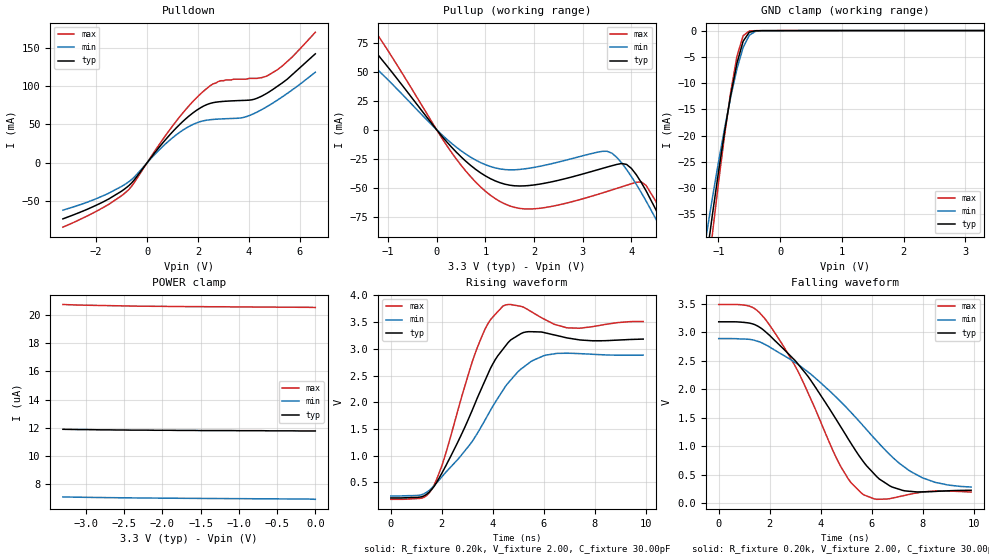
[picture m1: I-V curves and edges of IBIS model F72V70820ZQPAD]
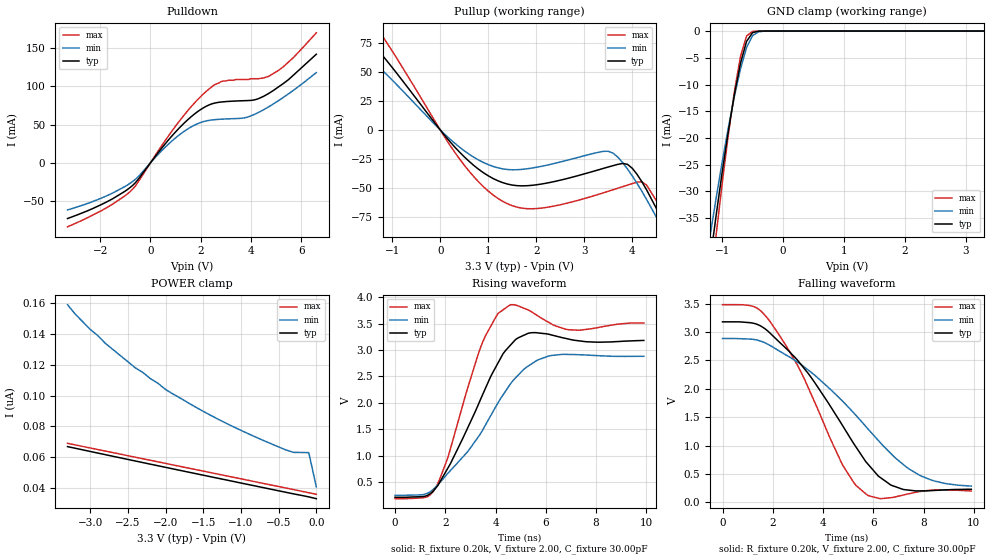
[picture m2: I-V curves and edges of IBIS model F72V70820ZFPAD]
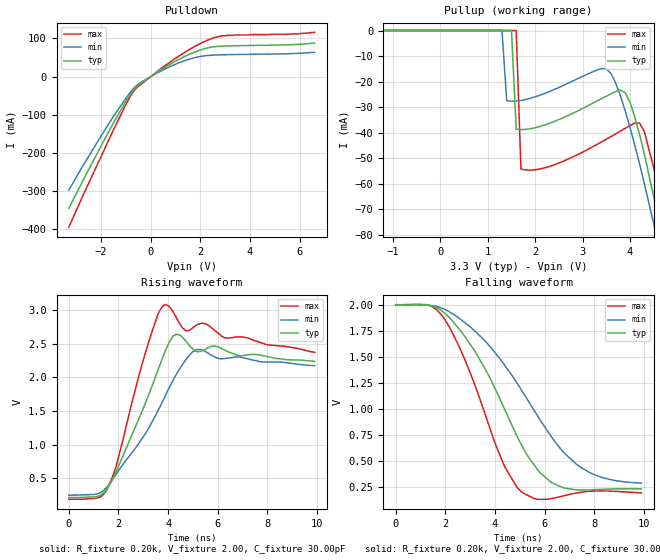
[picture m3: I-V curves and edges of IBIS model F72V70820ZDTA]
| IBIS file f72v7082.ibs created by s2ibis2 version 1.1
| North Carolina State University Electronics Research Laboratory  1995
[IBIS ver]   2.1
[File name]   f72v7082.ibs
[File Rev]   1.0
[Date]   02/03/2000
[Source]   Integrated Device Technology, Inc.
[Notes]   1. Temperatures: typ=25C, min=85C, max=-40C 2. Cemos9_3v
   process. 3. Ramp rates based on 50 ohm load.
[Copyright]   Copyright 1999, Integrated Device Technology, Inc.
|   Component idt72v70820z
[Component]   idt72v70820z
[Manufacturer]   Integrated Device Technology
[Package]
| variable   typ   min   max
R_pkg   0.75   0.60   0.90
L_pkg   8.10nH   8.30nH   9.90nH
C_pkg   0.53pF   0.46pF   0.60pF
[Pin]  signal_name   model_name   R_pin   L_pin   C_pin
1   GND   GND
2   VCC   POWER
3   TX8   F72V70820ZFPAD
4   TX9   F72V70820ZFPAD
5   TX10   F72V70820ZFPAD
6   TX11   F72V70820ZFPAD
7   TX12   F72V70820ZFPAD
8   TX13   F72V70820ZFPAD
9   TX14   F72V70820ZFPAD
10   TX15   F72V70820ZFPAD
11   GND   GND
12   RX0   F72V70820ZTTL2
13   RX1   F72V70820ZTTL2
14   RX2   F72V70820ZTTL2
15   RX3   F72V70820ZTTL2
16   RX4   F72V70820ZTTL2
17   RX5   F72V70820ZTTL2
18   RX6   F72V70820ZTTL2
19   RX7   F72V70820ZTTL2
20   RX8   F72V70820ZTTL2
21   RX9   F72V70820ZTTL2
22   RX10   F72V70820ZTTL2
23   RX11   F72V70820ZTTL2
24   RX12   F72V70820ZTTL2
25   RX13   F72V70820ZTTL2
26   RX14   F72V70820ZTTL2
27   RX15   F72V70820ZTTL2
28   F0I   F72V70820ZTTL
29   FE_HCLK   F72V70820ZTTL
30   GND   GND
31   CLK   F72V70820ZTTL
32   VCC   POWER
33   TMS   F72V70820ZTTLPU
34   TDI   F72V70820ZTTLPU
35   TDO   F72V70820ZFPAD
36   TCK   F72V70820ZTTL
37   TRST   F72V70820ZTTLU2
38   IC   F72V70820ZTTLPD
39   RESET   F72V70820ZTTL
40   WFPS   F72V70820ZTTL
41   A0   F72V70820ZTTL
42   A1   F72V70820ZTTL
43   A2   F72V70820ZTTL
44   A3   F72V70820ZTTL
45   A4   F72V70820ZTTL
46   A5   F72V70820ZTTL
47   A6   F72V70820ZTTL
48   A7   F72V70820ZTTL
49   DS_RD   F72V70820ZTTL
50   R_W_RW   F72V70820ZTTL
51   CS   F72V70820ZTTL
52   AS_ALE   F72V70820ZTTL
53   IM   F72V70820ZTTL
54   GND   GND
55   AD0   F72V70820ZQPAD
56   AD1   F72V70820ZQPAD
57   AD2   F72V70820ZQPAD
58   AD3   F72V70820ZQPAD
59   AD4   F72V70820ZQPAD
60   AD5   F72V70820ZQPAD
61   AD6   F72V70820ZQPAD
62   AD7   F72V70820ZQPAD
63   VCC   POWER
64   GND   GND
65   D8   F72V70820ZQPAD
66   D9   F72V70820ZQPAD
67   D10   F72V70820ZQPAD
68   D11   F72V70820ZQPAD
69   D12   F72V70820ZQPAD
70   D13   F72V70820ZQPAD
71   D14   F72V70820ZQPAD
72   D15   F72V70820ZQPAD
73   DTA   F72V70820ZDTA
74   CCO   F72V70820ZFPAD
75   GND   GND
76   ODE   F72V70820ZTTL
77   TX0   F72V70820ZFPAD
78   TX1   F72V70820ZFPAD
79   TX2   F72V70820ZFPAD
80   TX3   F72V70820ZFPAD
81   TX4   F72V70820ZFPAD
82   TX5   F72V70820ZFPAD
83   TX6   F72V70820ZFPAD
84   TX7   F72V70820ZFPAD
| Models and submodels in the file (8): F72V70820ZQPAD (I/O), F72V70820ZFPAD (3-state), F72V70820ZDTA (Output), F72V70820ZTTL (Input), F72V70820ZTTL2 (Input), F72V70820ZTTLPU (Input), F72V70820ZTTLU2 (Input), F72V70820ZTTLPD (Input)
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| FIN  FIN   dummy_model
| FOEL FOEL   dummy_model
| QIN  QIN   dummy_model
| QOEL QOEL   dummy_model
| DIN  DIN   dummy_model
|   Model F72V70820ZQPAD
[Model]   F72V70820ZQPAD
Model_type   I/O
Polarity   Non-Inverting
Enable   Active-Low
Vinl =  0.000V
Vinh =  3.000V
Vmeas =  1.500V
C_comp   3.00pF   NA   NA
[Temperature Range]   25.00   85.00   -40.00
[Voltage Range]   3.30V   3.00V   3.60V
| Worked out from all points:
|   slope of the pulldown table from 0 to 0.495 V, typ, clamps not added: 23.4 ohm
|   slope of the pullup table from 0 to 0.495 V, typ, clamps not added: 21.5 ohm
|   GND clamp passes 1 mA (typ) near -0.54 V on its own axis
|   rising waveform, R_fixture 0.20k, V_fixture 2.00, C_fixture 30.00pF: 20-80 % time 1.71ns typ, 2.27ns min, 1.23ns max; typ from 0.211 V to 3.18 V
|   falling waveform, R_fixture 0.20k, V_fixture 2.00, C_fixture 30.00pF: 20-80 % time 2.73ns typ, 3.51ns min, 2.12ns max; typ from 3.18 V to 0.229 V
[Pulldown]
| voltage   I(typ)   I(min)   I(max)
-3.3V     -72.9mA    -61.6mA    -83.7mA
-1.7V     -50.47mA   -42.52mA   -57.8mA
-800mV    -32mA      -26.54mA   -37.34mA
1.2V      47.35mA    37.83mA    56.6mA
1.9V      67.47mA    51.48mA    83.41mA
2.5V      77.67mA    56.26mA    101mA
2.9V      79.81mA    57.22mA    107mA
3.8V      81.36mA    59.3mA     109mA
4.2V      82.85mA    64.29mA    110mA
4.7V      90.6mA     73.15mA    113mA
5.3V      104mA      85.84mA    126mA
6.6V      142mA      118mA      170mA
[Pullup]
| voltage   I(typ)   I(min)   I(max)
-3.3V     146mA      105mA      190mA
-2.3V     116mA      90.88mA    147mA
-1.5V     79.72mA    63.5mA     100mA
-1V       53.96mA    43.07mA    68.21mA
400mV     -19.13mA   -14.87mA   -24.99mA
1.4V      -46.88mA   -34.3mA    -63.9mA
3.5V      -32.14mA   -18.54mA   -53.16mA
3.9V      -29.89mA   -34.29mA   -47.81mA
4.2V      -45.33mA   -54.06mA   -44.96mA
4.7V      -86.48mA   -93.01mA   -79.56mA
4.9V      -105mA     -110mA     -99.7mA
6.6V      -284mA     -270mA     -297mA
[GND_clamp]
| voltage   I(typ)   I(min)   I(max)
-3.3V     -263mA     -228mA     -298mA
-1.2V     -43.96mA   -39.28mA   -49.29mA
-1.1V     -35.25mA   -32mA      -38.93mA
-1V       -26.98mA   -25.08mA   -29.06mA
-900mV    -19.24mA   -18.57mA   -19.87mA
-800mV    -12.2mA    -12.56mA   -11.61mA
-700mV    -6.204mA   -7.29mA    -4.893mA
-600mV    -2.013mA   -3.2mA     -972uA
-500mV    -309uA     -878uA     -70.72uA
-400mV    -29.78uA   -143uA     -9.346uA
-300mV    -4.901uA   -18.95uA   -5.393uA
3.3V      11.76uA    6.916uA    20.55uA
[POWER_clamp]
| voltage   I(typ)   I(min)   I(max)
-3.3V     11.88uA    7.059uA    20.77uA
-3.1V     11.86uA    7.041uA    20.73uA
-2.3V     11.82uA    6.988uA    20.65uA
-1.7V     11.8uA     6.962uA    20.62uA
-1.5V     11.79uA    6.954uA    20.62uA
-1.1V     11.79uA    6.941uA    20.6uA
-1V       11.78uA    6.938uA    20.6uA
-700mV    11.78uA    6.928uA    20.59uA
-600mV    11.77uA    6.925uA    20.59uA
-500mV    11.77uA    6.922uA    20.58uA
-100mV    11.76uA    6.914uA    20.57uA
0V        11.76uA    6.89uA     20.56uA
[Ramp]
| variable   typ   min   max
dV/dt_r   1.29/1.36n   1.01/2.25n   1.57/0.87n
dV/dt_f   1.28/3.10n   1.01/4.05n   1.50/2.20n
R_load = 50.00
[Rising Waveform]
R_fixture = 0.20k
V_fixture = 2.00
C_fixture = 30.00pF
R_dut = 0.75
L_dut = 8.10nH
C_dut = 0.53pF
| time   V(typ)   V(min)   V(max)
0s        211mV      247mV      185mV
1.6ns     371mV      393mV      367mV
2ns       672mV      605mV      808mV
3.4ns     2.089V     1.424V     3.032V
3.9ns     2.626V     1.842V     3.539V
4.4ns     2.994V     2.226V     3.801V
5.2ns     3.305V     2.655V     3.78V
6.1ns     3.294V     2.883V     3.535V
7.4ns     3.167V     2.91V      3.385V
9.9ns     3.182V     2.882V     3.511V
[Falling Waveform]
R_fixture = 0.20k
V_fixture = 2.00
C_fixture = 30.00pF
R_dut = 0.75
L_dut = 8.10nH
C_dut = 0.53pF
| time   V(typ)   V(min)   V(max)
0s        3.18V      2.886V     3.483V
1.2ns     3.158V     2.873V     3.455V
1.9ns     2.98V      2.763V     3.182V
3.5ns     2.225V     2.301V     1.938V
4.8ns     1.331V     1.775V     634mV
5.6ns     775mV      1.392V     178mV
6.3ns     426mV      1.044V     72.11mV
7.2ns     229mV      663mV      130mV
8.5ns     209mV      367mV      215mV
9.9ns     229mV      286mV      198mV
|   Model F72V70820ZFPAD
[Model]   F72V70820ZFPAD
Model_type   3-state
Polarity   Non-Inverting
Enable   Active-Low
Vinl =  0.000V
Vinh =  3.000V
Vmeas =  1.500V
C_comp   3.00pF   NA   NA
[Temperature Range]   25.00   85.00   -40.00
[Voltage Range]   3.30V   3.00V   3.60V
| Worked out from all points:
|   slope of the pulldown table from 0 to 0.495 V, typ, clamps not added: 23.4 ohm
|   slope of the pullup table from 0 to 0.495 V, typ, clamps not added: 21.5 ohm
|   GND clamp passes 1 mA (typ) near -0.54 V on its own axis
|   rising waveform, R_fixture 0.20k, V_fixture 2.00, C_fixture 30.00pF: 20-80 % time 1.75ns typ, 2.28ns min, 1.25ns max; typ from 0.211 V to 3.18 V
|   falling waveform, R_fixture 0.20k, V_fixture 2.00, C_fixture 30.00pF: 20-80 % time 2.74ns typ, 3.51ns min, 2.14ns max; typ from 3.18 V to 0.229 V
[Pulldown]
| voltage   I(typ)   I(min)   I(max)
-3.3V     -72.8mA    -61.6mA    -83.7mA
-1.9V     -53.7mA    -45.35mA   -61.6mA
-800mV    -32.01mA   -26.54mA   -37.34mA
1.2V      47.36mA    37.84mA    56.62mA
1.9V      67.48mA    51.49mA    83.43mA
2.5V      77.68mA    56.27mA    101mA
2.9V      79.82mA    57.23mA    107mA
3.8V      81.36mA    59.3mA     109mA
4.2V      82.85mA    64.29mA    110mA
4.7V      90.6mA     73.15mA    113mA
5.3V      104mA      85.84mA    126mA
6.6V      142mA      118mA      170mA
[Pullup]
| voltage   I(typ)   I(min)   I(max)
-3.3V     146mA      106mA      190mA
-2.3V     116mA      90.89mA    147mA
-1.5V     79.73mA    63.51mA    100mA
-1V       53.97mA    43.08mA    68.23mA
400mV     -19.13mA   -14.87mA   -24.99mA
1.4V      -46.88mA   -34.3mA    -63.9mA
3.5V      -32.14mA   -18.51mA   -53.16mA
3.9V      -29.82mA   -33.81mA   -47.81mA
4.2V      -44.86mA   -53.11mA   -44.92mA
4.7V      -85.13mA   -91.19mA   -78.74mA
4.9V      -103mA     -108mA     -98.49mA
6.6V      -279mA     -265mA     -292mA
[GND_clamp]
| voltage   I(typ)   I(min)   I(max)
-3.3V     -257mA     -223mA     -293mA
-1.2V     -42.98mA   -38.32mA   -48.28mA
-1.1V     -34.44mA   -31.21mA   -38.11mA
-1V       -26.34mA   -24.44mA   -28.43mA
-900mV    -18.77mA   -18.08mA   -19.41mA
-800mV    -11.88mA   -12.22mA   -11.32mA
-700mV    -6.026mA   -7.079mA   -4.749mA
-600mV    -1.941mA   -3.095mA   -929uA
-500mV    -292uA     -843uA     -59.24uA
-400mV    -24.21uA   -135uA     -2.053uA
-300mV    -1.458uA   -16.11uA   -49.02nA
3.3V      33.11nA    63.46nA    33nA
[POWER_clamp]
| voltage   I(typ)   I(min)   I(max)
-3.3V     66.92nA    159nA      69.05nA
-3.2V     65.88nA    153nA      68.04nA
-3V       63.79nA    143nA      66.04nA
-2.9V     62.75nA    139nA      65.04nA
-2.8V     61.71nA    134nA      64.04nA
-2.4V     57.58nA    118nA      60.04nA
-1.9V     52.45nA    101nA      55.03nA
-1.3V     46.35nA    84.64nA    49.03nA
-700mV    40.28nA    70.88nA    43.02nA
-300mV    36.24nA    63.16nA    39.02nA
-100mV    34.31nA    63.03nA    37.01nA
0V        33.14nA    40.81nA    36.01nA
[Ramp]
| variable   typ   min   max
dV/dt_r   1.29/1.37n   1.01/2.24n   1.57/0.93n
dV/dt_f   1.28/3.10n   1.01/4.05n   1.50/2.21n
R_load = 50.00
[Rising Waveform]
R_fixture = 0.20k
V_fixture = 2.00
C_fixture = 30.00pF
R_dut = 0.75
L_dut = 8.10nH
C_dut = 0.53pF
| time   V(typ)   V(min)   V(max)
0s        211mV      247mV      185mV
1.6ns     375mV      396mV      376mV
2.1ns     761mV      664mV      962mV
3.5ns     2.171V     1.496V     3.163V
4.1ns     2.757V     2.003V     3.694V
4.5ns     3.044V     2.293V     3.831V
5.3ns     3.318V     2.696V     3.76V
6.2ns     3.289V     2.896V     3.502V
7.3ns     3.176V     2.912V     3.376V
9.9ns     3.182V     2.882V     3.513V
[Falling Waveform]
R_fixture = 0.20k
V_fixture = 2.00
C_fixture = 30.00pF
R_dut = 0.75
L_dut = 8.10nH
C_dut = 0.53pF
| time   V(typ)   V(min)   V(max)
0s        3.18V      2.886V     3.483V
1.2ns     3.158V     2.873V     3.455V
1.8ns     3.019V     2.786V     3.239V
3.1ns     2.441V     2.436V     2.316V
4.8ns     1.335V     1.772V     640mV
5.3ns     981mV      1.536V     300mV
5.7ns     716mV      1.337V     148mV
6.7ns     302mV      858mV      80.16mV
7.8ns     200mV      486mV      185mV
9.9ns     229mV      285mV      198mV
|   Model F72V70820ZDTA
[Model]   F72V70820ZDTA
Model_type   Output
Vmeas =  1.500V
C_comp   3.00pF   NA   NA
[Temperature Range]   25.00   85.00   -40.00
[Voltage Range]   3.30V   3.00V   3.60V
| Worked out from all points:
|   slope of the pulldown table from 0 to 0.495 V, typ, clamps not added: 23.4 ohm
|   rising waveform, R_fixture 0.20k, V_fixture 2.00, C_fixture 30.00pF: 20-80 % time 1.39ns typ, 1.93ns min, 902ps max; typ from 0.211 V to 2.23 V
|   falling waveform, R_fixture 0.20k, V_fixture 2.00, C_fixture 30.00pF: 20-80 % time 2.3ns typ, 3.02ns min, 1.73ns max; typ from 2 V to 0.227 V
[Pulldown]
| voltage   I(typ)   I(min)   I(max)
-3.3V     -345mA     -297mA     -394mA
-1.7V     -145mA     -124mA     -167mA
-1V       -64.57mA   -56.38mA   -72.75mA
-700mV    -35.55mA   -31.63mA   -39.13mA
-500mV    -22.44mA   -19.4mA    -25.6mA
400mV     17.24mA    14.26mA    20.09mA
1.2V      47.36mA    37.84mA    56.62mA
2V        69.73mA    52.76mA    86.75mA
2.6V      78.47mA    56.58mA    103mA
3.4V      80.84mA    57.89mA    109mA
5.5V      83.3mA     59.95mA    111mA
6.6V      87.77mA    63.64mA    116mA
[Pullup]
| voltage   I(typ)   I(min)   I(max)
-3.3V     66.93nA    154nA      70.31nA
1.3V      20.09nA    25nA       23.2nA
1.4V      19.09nA    -27.44mA   22.17nA
1.5V      18.09nA    -27.64mA   21.15nA
1.6V      -38.62mA   -27.6mA    20.12nA
1.7V      -38.76mA   -27.36mA   -54.17mA
3.4V      -26.67mA   -14.9mA    -43.57mA
3.8V      -23.33mA   -25.71mA   -39.32mA
4.2V      -40.6mA    -52.13mA   -36.17mA
4.5V      -65.11mA   -75.73mA   -53.81mA
4.9V      -103mA     -110mA     -93.8mA
6.6V      -289mA     -277mA     -300mA
[Ramp]
| variable   typ   min   max
dV/dt_r   1.11/1.39n   0.83/2.31n   1.38/0.89n
dV/dt_f   1.28/3.11n   1.01/4.06n   1.51/2.22n
R_load = 50.00
[Rising Waveform]
R_fixture = 0.20k
V_fixture = 2.00
C_fixture = 30.00pF
R_dut = 0.75
L_dut = 8.10nH
C_dut = 0.53pF
| time   V(typ)   V(min)   V(max)
0s        211mV      247mV      185mV
1.5ns     320mV      352mV      307mV
1.9ns     591mV      554mV      671mV
3.2ns     1.721V     1.231V     2.503V
3.8ns     2.311V     1.659V     3.065V
4.4ns     2.638V     2.087V     2.838V
4.7ns     2.545V     2.255V     2.694V
5.2ns     2.379V     2.413V     2.788V
5.9ns     2.462V     2.298V     2.69V
9.9ns     2.235V     2.174V     2.371V
[Falling Waveform]
R_fixture = 0.20k
V_fixture = 2.00
C_fixture = 30.00pF
R_dut = 0.75
L_dut = 8.10nH
C_dut = 0.53pF
| time   V(typ)   V(min)   V(max)
0s        2V         2V         2V
1.3ns     1.996V     1.997V     1.997V
1.9ns     1.934V     1.963V     1.885V
3.2ns     1.549V     1.743V     1.22V
4.4ns     988mV      1.415V     438mV
5.1ns     635mV      1.166V     194mV
6.2ns     303mV      754mV      130mV
7.3ns     219mV      461mV      189mV
8.4ns     224mV      331mV      207mV
9.9ns     227mV      283mV      190mV
